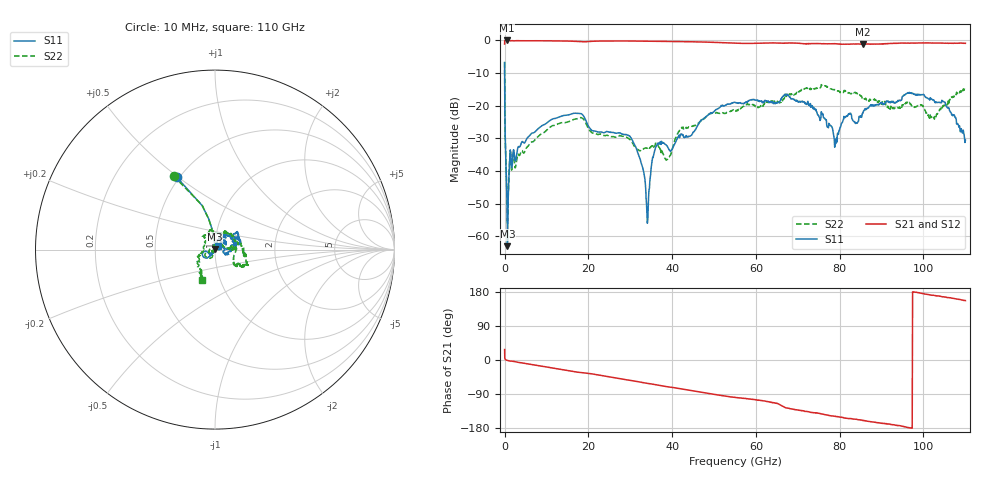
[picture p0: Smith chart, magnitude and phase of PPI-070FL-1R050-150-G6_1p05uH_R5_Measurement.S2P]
! Data measured by Modelithics Inc.  support@modelithics.com  813-866-6335  Tampa FL USA June 2025
! PPI-070FL-1R050-150-G6_1p05uH measured on 5-mil thick RO3003G2 board, mounted in 2-port shunt configuration on a 50-ohm transmission line
# GHz S RI R 50.0
!freq ReS11 ImS11 ReS21 ImS21 ReS12 ImS12 ReS22 ImS22
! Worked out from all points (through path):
!   1207 points, 10 MHz to 110 GHz, reference 50 ohm
!   highest |S21| = -0.01 dB at 494.2 MHz (marker M1); lowest = -1.2 dB at 85.6 GHz (marker M2)
!   group delay of S21, straight-line fit = 5.18 ps
!   lowest |S11| = -63.0 dB at 688.4 MHz (marker M3), VSWR 1.00, Z = 50 + j0.0655 ohm
!   |S11| at or under -10 dB: 16.29 MHz to end of sweep
!   |S22| runs from -56.1 to -6.6 dB; largest |S21 - S12| = 0.08
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0.01  -0.2138 0.4041  0.7789 0.4074  0.7789 0.4073  -0.2294 0.4093
0.2  -0.00172 0.0256  0.9979 0.0196  0.9978 0.0196  -0.00249 0.0257
0.4941776  -0.000479 0.00628  0.9986 -0.00815  0.9984 -0.00809  -0.00139 0.00634
0.6883552  -0.000266 0.000655  0.9981 -0.019  0.9981 -0.019  -0.00135 0.00079
1.756332  -0.00726 -0.00927  0.9895 -0.0563  0.9894 -0.0562  -0.00781 -0.00734
6.125328  -0.0205 -0.0294  0.9681 -0.1933  0.9682 -0.1929  -0.0112 -0.0243
18.35852  -0.0704 -0.0263  0.7969 -0.5288  0.7969 -0.5289  -0.0553 -0.0351
30.10626  -0.0248 -0.0212  0.575 -0.7923  0.5736 -0.7934  -0.0293 0.00129
32.63057  -0.00871 -0.00987  0.5065 -0.8359  0.5029 -0.838  -0.0102 0.0181
34.0869  -0.00146 0.000615  0.4639 -0.8581  0.4639 -0.8583  0.00291 0.0223
35.54323  0.00132 0.0172  0.4237 -0.8759  0.4189 -0.8784  0.0199 0.0114
36.7083  -7.74e-05 0.027  0.3878 -0.8894  0.3845 -0.8908  0.0242 0.000452
38.84425  -0.00465 0.0234  0.3219 -0.9097  0.3241 -0.9089  0.0143 0.00505
42.04818  0.0169 0.0327  0.2327 -0.9293  0.2286 -0.9303  0.0413 0.0188
55.05808  0.0791 0.0791  -0.1399 -0.8956  -0.133 -0.8966  0.084 0.00756
73.4  0.0961 0.00668  -0.6742 -0.5881  -0.6299 -0.6281  0.1542 -0.0883
79.1  0.0221 0.0143  -0.761 -0.4558  -0.733 -0.4977  0.1691 -0.0226
81.6  0.0602 0.0339  -0.7841 -0.3894  -0.747 -0.444  0.1596 -0.0288
85.6  0.0414 0.0678  -0.8186 -0.3055  -0.8094 -0.3338  0.1271 0.0336
91.7  0.0893 0.0727  -0.8768 -0.1764  -0.881 -0.1754  0.0332 0.085
104.6  0.1155 0.0234  -0.885 0.2122  -0.8871 0.1944  -0.0927 -0.0367
110  0.0195 0.0223  -0.8296 0.3587  -0.8319 0.3588  -0.0721 -0.1712
